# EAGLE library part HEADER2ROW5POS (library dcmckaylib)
2x5 0.1" header
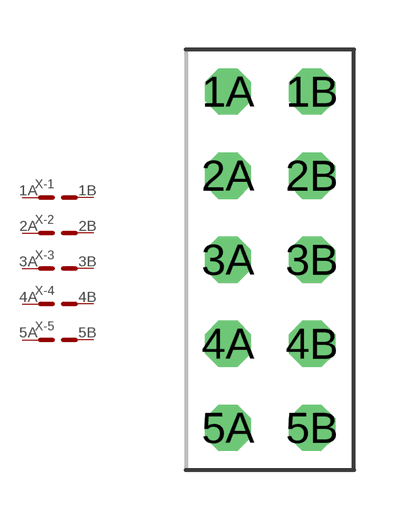
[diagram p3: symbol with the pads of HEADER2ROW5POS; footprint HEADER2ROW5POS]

Designator prefix X; gates -1=HEADER2ROW -2=HEADER2ROW -3=HEADER2ROW -4=HEADER2ROW -5=HEADER2ROW

## HEADER2ROW5POS  [HEADER2ROW5POS]
1A  -1:P$1
1B  -1:P$2
2A  -2:P$1
2B  -2:P$2
3A  -3:P$1
3B  -3:P$2
4A  -4:P$1
4B  -4:P$2
5A  -5:P$1
5B  -5:P$2

## Footprint HEADER2ROW5POS (pad centres in mm)
drill 0.889 octagon: 1A -1.27,5.08; 1B 1.27,5.08; 2A -1.27,2.54; 2B 1.27,2.54; 3A -1.27,0; 3B 1.27,0; 4A -1.27,-2.54; 4B 1.27,-2.54; 5A -1.27,-5.08; 5B 1.27,-5.08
